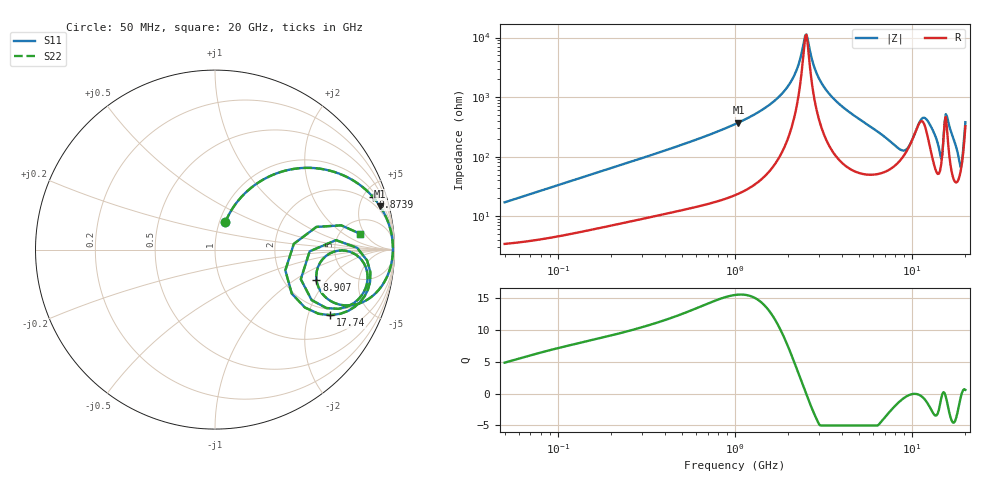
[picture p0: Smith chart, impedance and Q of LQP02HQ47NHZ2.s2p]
!Murata Part Number: LQP02HQ47NHZ2
!These Parameters are Measured in Series Mode Connection
!  o--[Z]--o
!Port1  Port2
!  o-------o
!Freq. Start=50[MHz] Stop=20[GHz], 401[Steps]
# Hz S RI R 50
!Freq.(Hz) S11(Real) S11(Imag) S21(Real) S21(Imag) S12(Real) S12(Imag) S22(Real) S22(Imag)
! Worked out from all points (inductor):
!   401 points, 50 MHz to 20 GHz, reference 50 ohm
!   read as one part in series: L = 53 nH near 51.52 MHz
!   highest Q = 15.6 at 1.046 GHz (marker M1), where L = 56.7 nH
!   self-resonance near 2.494 GHz
!   S11 on the Smith chart (normalised r, x): 50 MHz: 1.07, +0.34; 873.9 MHz: 1.39, +5.89; 8.907 GHz: 3.01, -1.54; 17.74 GHz: 1.74, -2.80; 20 GHz: 7.49, +3.91
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5e7  0.0579 0.1526  0.9421 -0.1526  0.9421 -0.1526  0.0579 0.1526
1.364002e8  0.1941 0.3383  0.8059 -0.3383  0.8059 -0.3383  0.1941 0.3383
3.721004e8  0.573 0.4523  0.427 -0.4523  0.427 -0.4523  0.573 0.4523
8.738837e8  0.8818 0.2916  0.1182 -0.2916  0.1182 -0.2916  0.8818 0.2916
1e9  0.911 0.2543  0.089 -0.2543  0.089 -0.2543  0.911 0.2543
1.045961e9  0.9196 0.2418  0.0804 -0.2418  0.0804 -0.2418  0.9196 0.2418
1.904239e9  0.9853 0.0759  0.0147 -0.0759  0.0147 -0.0759  0.9853 0.0759
2.211938e9  0.9903 0.0354  0.00974 -0.0354  0.00974 -0.0354  0.9903 0.0354
2.493527e9  0.9913 0.00281  0.00867 -0.00281  0.00867 -0.00281  0.9913 0.00281
2.728004e9  0.9904 -0.0219  0.00959 0.0219  0.00959 0.0219  0.9904 -0.0219
3.680849e9  0.9747 -0.108  0.0253 0.108  0.0253 0.108  0.9747 -0.108
7.442007e9  0.7162 -0.3101  0.2838 0.3101  0.2838 0.3101  0.7162 -0.3101
8.907419e9  0.5651 -0.1669  0.4349 0.1669  0.4349 0.1669  0.5651 -0.1669
1.019291e10  0.6843 -0.00622  0.3157 0.00622  0.3157 0.00622  0.6843 -0.00622
1.166392e10  0.8387 -0.0949  0.1613 0.0949  0.1613 0.0949  0.8387 -0.0949
1.314879e10  0.8156 -0.2572  0.1844 0.2572  0.1844 0.2572  0.8156 -0.2572
1.438523e10  0.5384 -0.2813  0.4616 0.2813  0.4616 0.2813  0.5384 -0.2813
1.504638e10  0.6738 0.0527  0.3262 -0.0527  0.3262 -0.0527  0.6738 0.0527
1.573793e10  0.8656 -0.1259  0.1344 0.1259  0.1344 0.1259  0.8656 -0.1259
1.774144e10  0.643 -0.3653  0.357 0.3653  0.357 0.3653  0.643 -0.3653
1.88369e10  0.3919 -0.1156  0.6081 0.1156  0.6081 0.1156  0.3919 -0.1156
2e10  0.8056 0.0896  0.1944 -0.0896  0.1944 -0.0896  0.8056 0.0896
